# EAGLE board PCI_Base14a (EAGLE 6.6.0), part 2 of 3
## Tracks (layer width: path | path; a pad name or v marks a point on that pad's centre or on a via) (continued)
CLK2  (via drill 0.3) (continued)
  Top 0.254: v31.75,124.45 32.07,124.45 32.07,114.45 31.75,114.13 31.75,109.68 30.48,108.41 30.48,107.62 30.32,107.46 30.32,81.9 29.69,81.27 29.69,72.38 v30,72.06 | v33.34,72.06 34.13,71.27 34.13,64.76 33.5,64.12 v33.5,59.36 | v68.58,60 68.9,60.31 68.9,69.2 v68.58,69.52 | v107.63,69.84 107.31,70.16 107.31,70.31 107,70.63 107,73.97 106.36,74.6 106.36,77.78 106.04,78.09 106.04,86.67 106.84,87.46 106.84,113.81 v107.16,114.13 | v103.82,114.13 104.14,114.45 104.14,138.89 v103.82,139.21
  Bottom 0.152: X6.J3-A27 arc-90 X6.J3-A27 100.33,139.21
  Bottom 0.254: v31.75,124.45 33.18,124.45 34.13,125.4 36.04,125.4 36.51,125.88 37.31,125.88 X2.B16 | v33.34,72.06 v30,72.06 | v33.5,59.36 33.81,59.68 34.92,59.68 35.56,60.31 36.67,60.31 36.99,60.63 46.35,60.63 47.47,59.52 48.74,59.52 49.21,60 v68.58,60 | v68.58,69.52 68.9,69.2 71.91,69.2 72.55,69.84 75.41,69.84 75.72,70.16 83.18,70.16 83.5,69.84 v107.63,69.84 | v103.82,114.13 v107.16,114.13 | 100.33,139.21 v103.82,139.21
CLK3  (via drill 0.3)
  Top 0.254: v7.46,126.04 7.46,127.15 8.1,127.78 8.1,142.7 7.78,143.02 7.78,150.8 7.46,151.12 v7.3,151.12 | v24.92,152.07 24.61,152.39 24.61,158.9 24.92,159.21 v24.92,167.15 | v73.34,166.68 73.34,156.36 73.66,156.04 73.66,150.17 73.34,149.85 73.34,147.15 74.93,145.56 74.93,142.39 73.82,141.28 v73.82,140.16
  Bottom 0.152: X6.J3-C27 89.38,139.21 88.74,139.93 88.15,140.2 81.36,140.2
  Bottom 0.254: v7.46,126.04 8.57,126.04 8.89,126.35 13.81,126.35 14.29,125.88 16.67,125.88 X3.B16 | v7.3,151.12 7.62,151.44 7.94,151.44 8.25,151.75 11.27,151.75 11.59,152.07 13.33,152.07 13.65,152.39 24.61,152.39 v24.92,152.07 | v24.92,167.15 26.51,167.15 26.83,166.83 27.62,166.83 27.94,166.52 48.58,166.52 49.21,167.15 49.85,167.15 50.96,166.04 63.82,166.04 64.45,166.68 v73.34,166.68 | v73.82,140.16 74.93,140.16 75.25,140.48 80.96,140.48 81.36,140.2
DEVSEL#  (via drill 0.3)
  Top 0.254: v85.25,109.21 84.93,108.89 84.93,106.67 84.61,106.35 84.61,101.11 84.93,100.79 84.93,89.84 85.25,89.52 85.25,84.13 84.14,83.01 v84.14,73.01 | v80.96,73.01 81.28,73.01 81.28,65.23 80.64,64.6 80.64,63.96 81.76,62.85 81.76,55.07 81.44,54.76 v81.44,53.65 | v29.37,58.09 v29.37,53.65 | v8.57,58.09 8.89,58.09 8.89,65.39 9.21,65.71 9.21,86.19 v8.89,86.51 | v20.48,87.94 20.64,88.09 20.64,88.25 21.43,89.05 22.38,89.05 23.34,90 23.65,90 23.97,90.32 24.92,90.32 25.4,90.79 v25.72,90.79 | v29.05,90.79 29.37,91.11 29.37,99.21 v29.05,99.52
  Bottom 0.152: X6.J3-D12 v85.25,109.21
  Bottom 0.254: 29.05,99.21 26.19,99.21 24.92,100.48 23.97,100.48 22.7,99.21 19.37,99.21 X3.B37 | 29.05,99.21 39.85,99.21 X2.B37 40,99.21 43.34,99.21 44.61,100.48 45.56,100.48 46.83,99.21 60.48,99.21 X1.B37 | v80.96,73.01 v84.14,73.01 | v81.44,53.65 81.12,53.96 39.69,53.96 39.37,53.65 v29.37,53.65 | v29.37,58.09 29.05,57.77 13.02,57.77 12.7,58.09 v8.57,58.09 | v8.89,86.51 17.3,86.51 18.57,87.78 20,87.78 20.16,87.94 v20.48,87.94 | v29.05,90.79 v25.72,90.79 | 29.05,99.21 v29.05,99.52
FRAME#  (via drill 0.3)
  Top 0.254: v10,101.43 10,98.57 10.32,98.25 10.32,88.25 10.64,87.94 10.64,64.76 10.32,64.44 10.32,57.14 10,56.82 v10,55.71 | v50.64,56.03 v50.64,61.27 50.64,72.22 v50.32,72.54 | v93.66,61.9 93.98,62.22 93.98,76.51 94.3,76.82 94.3,80.63 93.98,80.95 93.98,81.9 v94.14,82.06 | v99.22,82.06 98.9,82.38 98.9,88.41 99.22,88.73 99.22,89.36 98.9,89.68 98.9,97.62 99.22,97.94 99.22,98.57 98.11,99.68 98.11,109.53 98.42,109.84 v98.42,111.27 | v55.72,97.46 55.88,97.46 57.63,99.21 58.42,99.21 58.74,99.52 59.21,99.52 60.17,100.48 60.96,100.48 61.59,101.11 62.07,101.11 63.18,102.22 63.18,103.02 X1.A34 | v52.07,97.46 51.75,97.14 51.75,89.68 51.43,89.36 51.43,84.28 51.59,84.13 51.59,72.85 v51.91,72.54
  Bottom 0.152: X6.J3-A13 arc-90 93.42,111.27 v98.42,111.27
  Bottom 0.254: v10,101.43 16.03,101.43 16.35,101.75 17.3,101.75 18.57,103.02 21.75,103.02 X3.A34 21.91,103.02 24.92,103.02 25.24,102.7 26.03,102.7 26.51,102.22 36.51,102.22 36.99,101.75 37.94,101.75 39.21,103.02 42.39,103.02 X2.A34 | v10,55.71 11.11,55.71 11.43,56.03 13.02,56.03 13.33,56.34 31.27,56.34 31.59,56.66 45.88,56.66 46.2,56.34 49.05,56.34 49.37,56.03 v50.64,56.03 | v50.64,61.27 50.96,60.95 67.63,60.95 68.26,61.58 78.74,61.58 79.06,61.27 85.41,61.27 85.72,61.58 93.34,61.58 v93.66,61.9 | v99.22,82.06 v94.14,82.06 | v52.07,97.46 v55.72,97.46 | v50.32,72.54 v51.91,72.54
GND  (via drill 0.3)
  Top 0.254: X2.B57 40,73.97 40,74.44 40.16,74.6 42.54,74.6 42.54,75.08 X2.A56 42.54,75.24 42.54,75.87 43.81,77.14 43.81,80.63 43.66,80.79 43.66,82.7 43.5,82.86 43.5,83.17 42.54,84.13 42.54,85.24 X2.A48 | v35.88,83.97 v35.88,87.78 v35.88,97.94 v35.88,101.43 v35.88,103.02 v35.88,110.64 v35.88,118.26 | X3.A42 21.91,93.02 21.91,93.81 22.22,94.13 22.38,94.13 23.18,94.92 23.18,97.14 24.45,98.41 24.45,99.21 X3.A37 24.45,99.37 24.45,101.75 X3.A35 | v40.96,110.48 42.54,108.89 42.54,108.26 X2.A30 | X2.A24 42.54,115.88 42.54,116.51 v40.96,118.1 41.12,118.1 41.12,118.89 41.27,119.05 41.27,121.27 42.54,122.54 42.54,123.34 X2.A18 | X2.B17 40,124.77 40,127.15 X2.B15 40,127.31 40,129.69 X2.B13 | 40,130.32 37.62,130.32 37.46,130.48 37.46,130.96 X2.B12 | 40,130.32 40,129.85 X2.B13 | 40,130.32 40,130.64 42.07,130.64 42.39,130.96 X2.A12 | 40,130.32 X2.B13 | C3.2 51.12,143.5 v51.12,139.85 51.12,137.47 C4.2 51.12,137.31 v51.12,130.96 v51.12,129.69 | v59.05,140.16 60.64,141.75 60.64,142.39 X1.B3 | X1.B13 60.64,129.69 60.64,127.31 X1.B15 60.64,127.15 60.64,124.77 X1.B17 60.64,124.61 60.64,123.65 62.07,123.65 62.23,123.5 63.02,123.5 X1.A18 | v38.1,145.72 38.42,145.4 38.42,144.77 40,143.18 40,142.55 X2.B3 | v29.53,145.72 29.53,143.66 C1.2 29.53,143.5 29.53,137.47 C2.2 29.53,137.31 29.53,132.86 29.05,132.39 29.05,130.96 | X3.B17 19.37,124.77 19.37,127.15 X3.B15 19.37,127.31 19.37,129.69 X3.B13 | v15.24,130.96 v15.24,142.39 | v29.05,129.69 29.05,130.96 | v15.24,74.12 15.24,77.93 14.92,78.25 14.92,83.65 v15.24,83.97 v15.24,87.78 15.24,91.9 14.92,92.22 14.92,97.62 v15.24,97.94 v15.24,103.02 v15.24,110.64 v15.24,118.26 v15.24,124.61
  Top 0.254: v18.26,108.41 16.83,109.84 16.83,110.64 X3.B28 | 29.05,130.96 v29.37,130.96 | v76.83,35.07 76.83,38.09 C12.2 | 89.06,30.94 X7.16 89.06,30.79 | 89.06,34.91 X7.17 | 89.06,26.66 X7.15 | 95.57,8.4 JP4.1 | 89.06,18.09 X7.13 | v78.1,60.31 C8.- | v75.56,60.31 75.56,64.12 C7.+ | C10.- v86.36,60.31 86.36,64.12 C9.- v86.36,66.66 | v64.77,66.66 64.77,67.93 64.45,68.25 64.45,73.01 63.18,74.28 63.18,75.08 X1.A56 | X1.B46 58.1,87.78 58.1,86.98 60.64,84.44 60.64,84.28 60.48,84.13 X1.B49 | v47.47,98.41 47.15,98.1 47.15,92.86 v47.47,92.86 47.47,92.54 47.62,92.38 47.62,91.27 48.1,90.79 48.1,88.89 48.42,88.57 48.42,88.41 v48.58,88.25 | X2.A35 45.08,101.75 45.08,99.37 X2.A37 | X1.A42 63.18,93.02 63.18,93.81 64.45,95.08 64.45,97.14 65.72,98.41 65.72,99.21 X1.A37 65.72,99.37 65.72,101.75 X1.A35 | v56.51,118.26 v56.51,110.64 | v61.59,118.1 63.18,116.51 63.18,115.88 X1.A24 | 71.12,108.41 71.12,115.56 C16.2 | 71.12,108.41 71.12,108.1 C15.2 | 71.12,108.41 v69.85,108.41 | 71.12,108.41 C15.2 | v61.59,110.48 63.18,108.89 63.18,108.26 X1.A30 | C15.2 71.12,107.94 v71.12,101.75 v71.12,100 | H1.B3,3 87.79,153.18 87.79,147.31 87.31,146.83 87.31,145.24 X6.J3-D30 | C17.2 96.52,79.52 96.52,81.11 96.04,81.59 96.04,86.82 v96.36,87.14 96.04,86.98 96.04,91.75 v96.36,92.06 96.04,91.9 96.04,94.92 v96.36,95.24 | 83.66,100.48 v83.66,107.3 v83.62,110.24 83.94,110.56 83.98,114.92 v83.66,115.24 v83.7,118.14 83.82,118.26 v83.82,125.24 84.14,125.24 84.14,129.85 v83.9,130.2 84.14,130 84.14,133.97 84.45,134.29 v84.45,135.24 v84.45,138.26 83.82,138.89 v83.82,145.24 | v94.77,105.24 v94.77,112.22 v94.77,113.18
  Top 0.254: v94.77,122.23 v94.77,125.24 95.09,125.56 v95.09,132.07 v95.09,133.18 94.77,133.5 94.77,136.51 95.09,136.83 95.09,140.96 v94.77,141.28 | C5.2 71.44,143.5 71.44,137.47 C6.2 71.44,137.31 v71.44,135.08 v71.44,129.69 | v83.66,95.24 83.34,95.56 83.34,100.16 83.66,100.48 | 83.66,100.48 v83.7,100.2 | v93.34,79.52 93.34,87.14 X6.J3-A1 | v87.79,64.28 87.79,79.52 H2.B3,3 | v80.17,35.07 80.49,35.39 v80.49,57.93
  Top 0.813: 89.06,34.91 89.06,30.94 | 89.06,26.66 89.06,30.79 | v95.57,16.34 95.57,8.4 | 89.06,18.09 v89.06,16.34 | v86.36,18.24 v86.36,26.66 | v76.68,10.94 v76.68,18.24
  Bottom 0.152: X6.J3-A1 93.36,87.14 v96.36,87.14 101.6,87.14 | X6.J3-D30 87.36,145.24 v83.82,145.24 80.01,145.24 | X6.J3-D27 87.36,139.05 83.66,139.05 80.01,139.05 | X6.J3-C26 88.8,138.1 arc90 88.65,138.26 v84.45,138.26 83.66,138.26 81.44,138.26 | X6.J3-D20 87.36,125.24 | 87.36,125.24 87.63,125.24 | 87.36,125.24 v83.82,125.24 80.01,125.24 | X6.J3-D11 87.36,107.3 v83.66,107.3 79.85,107.3 | X6.J3-D5 87.36,95.24 v83.66,95.24 80.01,95.24 | X6.J3-C4 88.57,94.29 83.66,94.13 81.28,94.13 | X6.J3-A28 arc-90 93.43,141.28 v94.77,141.28 100.17,141.28 | X6.J3-A20 arc90 93.49,125.08 100.17,125.08 | X6.J3-A14 arc90 93.55,113.02 100.33,113.02 | X6.J3-A10 93.36,105.18 arc90 93.61,104.92 97,104.92 100.33,104.92 | X6.J3-A5 arc-90 93.39,95.24 v96.36,95.24 100.17,95.24 | X6.J3-C22 89.36,129.91 arc66 88.49,130.14 arc24 88.31,130.2 v83.9,130.2 | v83.9,130.2 81.28,130.16 | X6.J3-C16 89.36,117.84 arc90 88.47,118.22 v83.7,118.14 81.28,118.1 | X6.J3-C12 89.36,110.07 arc19 88.47,110.19 arc71 88.51,110.2 v83.62,110.24 81.28,110.32 | X6.J3-C7 89.36,99.91 arc90 88.47,100.2 v83.7,100.2 81.28,100.16 | X6.J3-D15 arc90 87.33,115.24 v83.66,115.24 80.01,115.24 | X6.J3-B18 91.36,121.97 arc-90 91.61,122.23 v94.77,122.23 101.6,122.23 | X6.J3-B23 91.36,131.81 arc-90 91.61,132.07 92.23,132.07 92.23,132.31 94.06,132.23 94.06,132.07 v95.09,132.07 101.6,132.07 | X6.J3-A24 arc90 93.39,133.18 v95.09,133.18 100.33,133.18 | X6.J3-D25 arc90 87.33,135.24 v84.45,135.24 80.17,135.24 | X6.J3-B9 92.47,103.87 arc-90 92.72,104.29 97,104.29 101.6,104.13 | X6.J3-B13 92.23,111.97 arc-90 92.65,112.22 v94.77,112.22 101.44,112.14
  Bottom 0.152: X6.J3-B3 91.36,91.81 arc-56 91.47,92.02 arc-34 91.61,92.22 94.69,92.22 94.69,92.06 v96.36,92.06 101.6,92.06 | 86.36,129.53 86.27,129.53 | 78.42,129.85 78.5,129.81 | 78.9,130 78.91,129.98 | 67.47,128.58 67.46,128.6 | 66.52,128.89 66.51,128.82 | 65.88,129.58 65.88,129.53 X1.A13 65.88,129.69 | 80.01,131.12 80.01,131.15 | 77.47,131.75 77.47,131.72 | 77.31,131.75 77.31,131.72 | 80.64,131.75 80.64,131.72 | 72.55,129.21 72.54,129.27 | 72.87,129.53 72.91,129.48 | 76.68,129.37 76.69,129.47 | 75.25,129.21 75.25,129.24 | 66.83,129.21 66.87,129.18 | 86.84,130.16 86.83,130.21 | 80.17,129.53 80.27,129.51 | 78.1,129.21 78.1,129.24 | 69.21,128.1 69.21,128.13 | 69.53,128.1 69.45,128.13 | 67.79,128.58 67.79,128.68 | 83.66,130.32 v83.9,130.2 | 80.33,131.12 80.33,131.22 | 77.79,130.64 77.84,130.74 | 77.63,130.64 77.59,130.72 | 72.71,130.8 72.66,130.69 | 72.87,130.8 72.81,130.77 | 73.66,130.48 73.66,130.51 | 78.26,131.75 78.26,131.72 | 80.01,131.75 80.01,131.72 | 72.23,130.64 72.24,130.74 72.23,130.8 | 71.6,130 v71.44,129.69 71.6,129.85 | 74.61,129.53 74.61,129.5 | 76.36,129.53 76.36,129.5 | 72.39,130.8 72.39,130.74 | 67.63,128.58 67.64,128.68 | 83.34,130.48 83.35,130.45 | 86.68,130.48 86.62,130.42 | 69.53,128.26 69.54,128.36 | 66.83,128.42 66.87,128.46 | 73.98,130.96 73.97,130.86 | 80.96,130.16 80.95,130.06 | 80.64,129.85 80.66,129.82 | 78.9,131.27 79,131.26 | 70.33,130.8 70.33,130.77 | 72.07,130.8 72.12,130.69 | 73.5,130.48 73.5,130.51 | 73.98,131.75 73.97,131.69 | 70.64,130.8 70.64,130.77 | S2.2
  Bottom 0.254: v35.88,87.78 37.31,87.78 X2.B46 | v35.88,83.97 35.88,83.65 37.46,83.65 37.78,83.97 39.69,83.97 39.85,84.13 | 39.85,84.13 40.16,84.44 40.64,84.44 41.43,85.24 42.39,85.24 X2.A48 | 39.85,84.13 X2.B49 | v35.88,97.94 37.31,97.94 X2.B38 | v35.88,103.02 37.31,103.02 X2.B34 | v35.88,110.64 37.31,110.64 X2.B28 37.46,110.64 40.48,110.64 40.64,110.48 v40.96,110.48 | v35.88,118.26 37.31,118.26 X2.B22 37.46,118.26 40.48,118.26 40.64,118.1 v40.96,118.1 | v35.88,101.43 35.56,101.75 24.45,101.75 X3.A35 | X2.A12 42.54,130.96 43.18,130.96 44.45,129.69 44.93,129.69 X2.A13 45.08,129.69 v51.12,129.69 | X2.A18 42.39,123.34 41.91,123.34 40.64,124.61 40,124.61 X2.B17 | v59.05,140.16 58.74,140.16 58.42,139.85 v51.12,139.85 | 58.98,130.56 59.85,129.69 60.48,129.69 X1.B13 | 58.98,130.56 58.58,130.96 58.1,130.96 X1.B12 57.94,130.96 v51.12,130.96 | 58.98,130.56 59.05,130.64 61.59,130.64 61.91,130.96 63.02,130.96 X1.A12 63.18,130.96 63.98,130.96 64.29,130.64 64.77,130.64 65.56,129.85 X1.A13 65.72,129.69 65.88,129.69 v71.44,129.69 | v38.1,145.72 37.78,145.4 29.84,145.4 v29.53,145.72 | X3.A18 21.75,123.5 20.95,124.29 20.48,124.29 20.16,124.61 19.37,124.61 X3.B17 19.21,124.61 v15.24,124.61 | 17.7,130.56 18.57,129.69 19.21,129.69 X3.B13 | 17.7,130.56 17.3,130.96 16.83,130.96 X3.B12 16.67,130.96 v15.24,130.96 | v15.24,142.39 19.21,142.39 X3.B3 | 17.7,130.56 17.78,130.64 20.48,130.64 20.8,130.96 21.75,130.96 X3.A12 21.91,130.96 22.54,130.96 23.81,129.69 24.29,129.69 X3.A13 24.45,129.69 v29.05,129.69 | X3.A56 21.75,75.08 21.11,75.08 19.84,73.81 19.37,73.81 X3.B57 19.21,73.81 16.35,73.81 16.03,74.12 v15.24,74.12
  Bottom 0.254: v15.24,87.78 16.67,87.78 X3.B46 | v15.24,83.97 15.24,83.65 16.99,83.65 17.3,83.97 19.05,83.97 19.21,84.13 X3.B49 19.37,84.13 19.68,84.44 20,84.44 20.8,85.24 21.75,85.24 X3.A48 | v15.24,97.94 16.67,97.94 X3.B38 | v15.24,103.02 16.67,103.02 X3.B34 | v15.24,110.64 16.67,110.64 X3.B28 | v15.24,118.26 16.67,118.26 X3.B22 16.83,118.26 17.78,118.26 17.78,116.83 18.89,115.72 21.75,115.72 X3.A24 | v18.26,108.41 18.57,108.41 18.89,108.1 21.75,108.1 X3.A30 | v29.37,130.96 37.31,130.96 X2.B12 | v76.83,35.07 v80.17,35.07 83.5,35.07 X7.7 83.66,35.07 | 83.66,26.66 X7.5 | 89.06,26.66 X7.15 | 89.06,35.07 X7.17 | 83.66,18.24 X7.3 83.5,18.24 | 89.06,18.24 X7.13 | 74.93,10.94 X5.1 | v75.56,60.31 v78.1,60.31 v86.36,60.31 | X1.B57 60.64,73.81 61.44,73.81 62.71,75.08 63.02,75.08 X1.A56 | v64.77,66.66 65.09,66.35 76.99,66.35 77.31,66.66 v86.36,66.66 | X1.A48 63.02,85.24 61.75,85.24 60.8,84.28 60.64,84.28 60.48,84.13 X1.B49 | v47.47,92.86 42.54,92.86 X2.A42 | X2.A37 45.08,99.21 46.04,99.21 46.51,98.73 47.15,98.73 v47.47,98.41 47.31,98.73 55.56,98.73 56.36,97.94 57.94,97.94 X1.B38 58.1,97.94 60.96,97.94 61.59,98.57 62.07,98.57 62.71,99.21 65.56,99.21 X1.A37 | v48.58,88.25 48.89,88.57 55.56,88.57 56.36,87.78 57.94,87.78 X1.B46 | X1.B34 58.1,103.02 61.12,103.02 61.75,102.38 62.07,102.38 62.71,101.75 65.56,101.75 X1.A35 65.72,101.75 v71.12,101.75 | v56.51,110.64 57.94,110.64 X1.B28 58.1,110.64 61.12,110.64 61.28,110.48 v61.59,110.48 | v56.51,118.26 57.94,118.26 X1.B22 58.1,118.26 61.12,118.26 61.28,118.1 v61.59,118.1 | v69.85,108.41 66.36,108.41 66.04,108.1 63.18,108.1 X1.A30 | 83.66,94.13 v83.66,95.24
  Bottom 0.254: X6.J3-C4 89.38,93.17 89.85,93.17 90.96,92.06 91.44,92.06 91.47,92.02 | 97,104.29 97,104.92 | v94.77,105.24 93.5,105.24 X6.J3-A10 | v94.77,113.18 93.5,113.18 X6.J3-A14 | X6.J3-B13 91.28,111.11 90.96,110.8 90.49,110.8 89.85,110.16 89.38,110.16 88.47,110.19 | v94.77,125.24 93.5,125.24 X6.J3-A20 | 83.66,138.26 83.66,139.05 | v71.44,135.08 71.75,134.77 79.69,134.77 80.17,135.24 | X6.J3-B23 91.28,131.12 90.96,130.8 90.49,130.8 89.85,130.16 89.22,130.16 88.49,130.14 | v93.34,79.52 H2.B3,3 | v71.12,100 74.14,100 74.45,99.68 80.8,99.68 81.28,100.16 | v87.79,64.28 86.52,64.28 C9.- | v80.49,57.93 78.26,57.93 C8.- | S2.2 109.38,8.4 111.12,10.15 111.12,119.76 110.65,120.24 108.97,120.24 JP5.2
  Bottom 0.813: 89.06,26.66 v86.36,26.66 83.66,26.66 | 89.06,35.07 83.66,35.07 | v89.06,16.34 v95.57,16.34 | 89.06,18.24 v86.36,18.24 83.66,18.24 | v76.68,18.24 83.5,18.24 | 74.93,10.94 v76.68,10.94
  other vias: 27.94,100.95 27.78,107.94 27.62,112.86 9.84,106.19 101.28,111.27
  pour Top (isolate 0.254): -1.27,188.74 115.57,188.74 115.57,-1.76 -1.27,-1.76
  pour Bottom (isolate 0.254): -1.27,188.74 115.57,188.74 115.57,-1.76 -1.27,-1.76
GNT1#  (via drill 0.3)
  Top 0.254: v79.53,146.36 v79.53,124.61 | v88.42,146.2 91.44,149.21 v91.44,150.8 | v102.08,152.07 102.08,148.26 101.12,147.31 101.12,135.4 v101.44,135.08
  Bottom 0.152: X6.J3-A25 arc90 93.49,135.08 100.17,135.08
  Bottom 0.254: v79.53,124.61 65.72,124.61 X1.A17 | v79.53,146.36 87.79,146.36 87.95,146.2 v88.42,146.2 | v91.44,150.8 96.84,150.8 97.47,151.44 99.06,151.44 99.38,151.75 100.17,151.75 100.49,152.07 v102.08,152.07 | 100.17,135.08 v101.44,135.08
GNT2#  (via drill 0.3)
  Top 0.254: v55.56,124.61 55.56,125.88 55.24,126.19 55.24,133.81 55.88,134.45 57.31,134.45 57.63,134.77 58.42,134.77 v59.53,135.88 | v78.74,136.2 v78.74,133.5
  Bottom 0.152: X6.J3-C25 89.36,136.05 arc90 89.22,136.2 81.28,136.2
  Bottom 0.254: v55.56,124.61 45.08,124.61 X2.A17 | v59.53,135.88 60.01,135.88 60.17,136.04 61.12,136.04 61.75,135.4 62.07,135.4 62.71,134.77 63.66,134.77 64.29,134.13 64.61,134.13 65.25,133.5 67.63,133.5 67.94,133.81 78.42,133.81 v78.74,133.5 | 81.28,136.2 v78.74,136.2
GNT3#  (via drill 0.3)
  Top 0.254: v27.62,124.45 27.3,124.77 27.3,130.8 27.62,131.12 27.62,131.75 27.15,132.23 27.15,139.85 26.99,140.01 26.99,149.21 27.78,150.01 27.78,150.96 26.99,151.75 26.99,157.31 27.3,157.63 27.3,162.07 26.99,162.39 v26.99,165.56 | v64.77,165.88 64.93,165.72 64.93,165.09 65.25,164.77 65.25,157.94 66.04,157.15 v66.04,146.67
  Bottom 0.152: X6.J3-C30 89.36,146.83 80.17,146.83 80.01,146.83
  Bottom 0.254: v27.62,124.45 27.46,124.61 24.45,124.61 X3.A17 | v26.99,165.56 64.45,165.56 v64.77,165.88 | v66.04,146.67 78.74,146.67 79.22,147.15 79.85,147.15 80.17,146.83
IDSEL1  (via drill 0.3)
  Top 0.254: v69.06,113.81 68.74,113.81 68.74,118.26 69.06,118.57 69.06,121.91 v69.37,122.23
  Bottom 0.152: X6.J3-C18 89.36,121.97 arc90 89.11,122.23 81.28,122.23
  Bottom 0.254: v69.06,113.81 66.67,113.81 66.04,113.18 63.18,113.18 X1.A26 | 81.28,122.23 v69.37,122.23
IDSEL2  (via drill 0.3)
  Top 0.254: v47.47,120.32 47.15,120 47.15,116.51 46.67,116.03 46.67,114.29 45.56,113.18 44.61,113.18 43.81,113.97 42.7,113.97 42.54,113.81 42.54,113.34 X2.A26 | v52.23,136.04 v52.23,120.32 | v64.13,137.62 64.13,137.94 64.45,138.26 64.45,140.32 65.25,141.12 66.04,141.12 66.36,141.43 v66.67,141.43 | v72.23,138.74 v72.23,141.59 | v72.55,136.04 72.55,130.96 73.18,130.32 73.18,129.69 72.87,129.37 72.87,121.75 v73.18,121.43
  Bottom 0.152: X6.J3-D18 87.36,121.27 80.01,121.27
  Bottom 0.254: v47.47,120.32 47.78,120 51.91,120 v52.23,120.32 | v52.23,136.04 53.02,136.83 57.15,136.83 57.63,137.31 58.42,137.31 59.05,137.94 59.53,137.94 60.17,138.58 61.12,138.58 61.75,137.94 62.07,137.94 62.71,137.31 63.5,137.31 63.82,137.62 v64.13,137.62 | v66.67,141.43 67.15,141.43 67.31,141.59 v72.23,141.59 | v72.23,138.74 72.55,138.42 v72.55,136.04 | v73.18,121.43 73.5,121.75 79.53,121.75 80.01,121.27
IDSEL3  (via drill 0.3)
  Top 0.254: v23.02,114.76 22.86,114.76 21.91,113.81 21.91,113.34 X3.A26 | v34.29,113.65 34.29,120.64 34.61,120.96 34.61,127.94 33.34,129.21 33.34,134.29 33.5,134.45 33.5,135.08 33.18,135.4 33.18,137.78 34.13,138.74 34.13,142.07 34.45,142.39 34.45,147.31 33.81,147.94 33.81,153.66 34.29,154.13 v34.29,164.45 | v65.72,165.41 65.72,158.26 66.52,157.47 66.52,147.94 67.47,146.99 67.47,142.7 v67.15,142.39 | v86.04,141.59 85.72,141.28 85.72,134.93 86.2,134.45 86.2,132.54 85.57,131.91 85.57,125.24 87.31,123.5 87.31,123.34 X6.J3-D19
  Bottom 0.152: X6.J3-D19 87.36,123.18
  Bottom 0.254: v23.02,114.76 23.97,115.72 25.88,115.72 27.62,113.97 33.97,113.97 v34.29,113.65 | v34.29,164.45 34.61,164.14 36.35,164.14 36.67,163.82 42.54,163.82 42.86,164.14 45.24,164.14 46.2,165.09 65.4,165.09 v65.72,165.41 | v67.15,142.39 67.47,142.07 71.6,142.07 72.07,142.55 80.49,142.55 81.6,141.43 85.88,141.43 v86.04,141.59
INTA#  (via drill 0.3)
  Top 0.254: v23.02,144.61 23.02,144.29 23.18,144.13 23.18,140.64 21.91,139.37 21.91,138.74 X3.A6 | v24.13,159.53 v24.13,146.36 | v66.52,158.9 66.67,158.74 66.67,158.1 66.99,157.79 66.99,148.26 67.94,147.31 67.94,141.12 v67.63,140.8 | v45.88,143.66 44.61,143.66 43.81,142.86 43.81,140.64 42.54,139.37 42.54,138.74 X2.A6 | v56.04,144.13 55.72,144.45 55.72,152.07 56.04,152.39 56.04,153.18 56.36,153.5 v56.36,158.9 | v97.15,159.21 v97.15,144.21
  Bottom 0.152: v97.15,144.21 92.31,144.21 X6.J3-B29
  Bottom 0.254: v23.02,144.61 23.02,145.24 v24.13,146.36 | v24.13,159.53 24.45,159.21 33.65,159.21 34.29,158.58 56.36,158.58 | 56.36,158.58 66.2,158.58 v66.52,158.9 66.83,159.21 v97.15,159.21 | v67.63,140.8 68.1,140.32 68.1,139.05 66.52,139.05 66.04,138.58 63.18,138.58 X1.A6 | v45.88,143.66 46.67,144.45 55.72,144.45 v56.04,144.13 | 56.36,158.58 v56.36,158.9
INTB#  (via drill 0.3)
  Top 0.254: X1.B7 60.64,137.47 60.64,137.62 58.74,137.62 58.42,137.31 57.63,137.31 56.51,138.42 v56.51,138.58 56.2,138.89 56.2,143.18 56.83,143.82 56.83,144.13 57.31,144.61 v57.31,146.51 | v70.96,144.93 70.64,145.24 70.64,150.01 70.96,150.32 70.96,161.75 71.28,162.07 v71.28,163.82 | v52.23,146.51 v52.23,163.82
  Bottom 0.152: X6.J3-C29 88.65,143.8 arc90 87.84,144.21 85.09,144.21 85.09,144.29 81.44,144.37
  Bottom 0.254: v56.51,138.58 56.2,138.89 52.07,138.89 51.75,138.58 44.61,138.58 43.97,137.94 43.66,137.94 43.02,137.31 40,137.31 X2.B7 39.85,137.31 36.99,137.31 36.51,136.83 33.65,136.83 32.07,135.24 28.26,135.24 24.92,138.58 23.97,138.58 23.34,137.94 23.02,137.94 22.38,137.31 19.37,137.31 X3.B7 | 81.44,144.37 80.96,144.77 77.79,144.77 77.47,145.09 73.18,145.09 72.87,144.77 71.12,144.77 v70.96,144.93 | v71.28,163.82 70.96,164.14 52.55,164.14 v52.23,163.82 | v57.31,146.51 v52.23,146.51
INTC#  (via drill 0.3)
  Top 0.254: v69.69,137.31 69.37,137.62 69.37,142.7 v69.69,143.02 69.37,142.86 69.37,147.63 69.69,147.94 v69.69,150.96 | v26.03,150.17 26.03,139.69 24.92,138.58 24.76,138.58 24.45,138.26 24.45,137.47 X3.A7 | v46.67,150.17 46.67,139.69 45.08,138.1 45.08,137.47 X2.A7
  Bottom 0.152: X6.J3-D29 87.36,143.02 80.01,143.02
  Bottom 0.254: v69.69,137.31 65.72,137.31 X1.A7 | 80.01,143.02 v69.69,143.02 | v26.03,150.17 26.35,149.85 43.02,149.85 43.34,150.17 v46.67,150.17 46.99,149.85 51.59,149.85 52.7,150.96 53.34,150.96 53.97,150.32 63.34,150.32 63.66,150.64 69.37,150.64 v69.69,150.96
INTD#  (via drill 0.3)
  Top 0.254: v14.45,136.04 14.76,136.35 14.76,141.75 14.45,142.07 v14.45,149.37 | v35.08,136.04 35.08,141.43 35.4,141.75 35.4,148.26 v35.08,148.58 35.4,148.42 35.4,151.59 35.08,151.91 v35.08,153.02 | v55.09,136.04 54.77,136.35 v54.77,153.02 | v103.5,158.42 v103.5,142.23 | v75.88,153.18 v75.88,157.47
  Bottom 0.152: 101.6,142.15 92.47,142.23 X6.J3-B28
  Bottom 0.254: v14.45,136.04 16.67,136.04 X3.B8 | v14.45,149.37 21.91,149.37 22.7,148.58 23.34,148.58 23.65,148.9 34.77,148.9 v35.08,148.58 | v35.08,136.04 37.31,136.04 X2.B8 | v55.09,136.04 57.94,136.04 X1.B8 | v35.08,153.02 36.19,153.02 36.51,152.71 47.62,152.71 47.94,153.02 v54.77,153.02 55.88,153.02 56.04,153.18 57.78,153.18 58.42,153.82 71.91,153.82 72.23,153.5 75.88,153.5 v75.88,153.18 | v103.5,142.23 101.6,142.15 | v103.5,158.42 96.84,158.42 96.52,158.74 78.58,158.74 77.31,157.47 v75.88,157.47
IRDY#  (via drill 0.3)
  Top 0.254: v17.94,103.97 19.37,102.54 19.37,101.91 X3.B35 | v9.21,103.97 9.21,101.11 9.52,100.79 9.52,98.25 9.84,97.94 9.84,87.94 10.16,87.62 10.16,65.08 9.84,64.76 9.84,57.46 9.52,57.14 9.52,56.34 9.21,56.03 v9.21,54.92 | v51.43,55.23 51.43,62.22 51.12,62.54 51.12,83.81 50.96,83.97 50.96,89.68 51.28,90 v51.28,102.06 | v82.87,112.22 82.87,106.99 83.18,106.67 83.18,100.79 82.87,100.48 82.87,92.86 83.18,92.54 83.18,76.98 v82.87,76.66 | v79.53,67.46 v79.53,76.35 | v65.72,67.14 65.56,66.98 65.56,66.35 65.25,66.03 65.25,58.88 65.56,58.57 v65.56,55.23
  Bottom 0.152: X6.J3-C13 89.36,111.97 arc90 89.11,112.22 v82.87,112.22
  Bottom 0.254: v17.94,103.97 17.62,103.97 17.3,104.29 16.35,104.29 16.03,103.97 v9.21,103.97 | v9.21,54.92 10.32,54.92 10.64,55.23 11.43,55.23 11.75,55.55 13.33,55.55 13.65,55.87 31.59,55.87 31.91,56.19 45.56,56.19 45.88,55.87 48.74,55.87 49.05,55.55 50.01,55.55 50.32,55.23 v51.43,55.23 51.75,54.92 65.25,54.92 v65.56,55.23 | X1.B35 60.48,101.75 51.59,101.75 v51.28,102.06 51.43,101.75 48.58,101.75 48.42,101.91 46.67,101.91 45.56,103.02 44.61,103.02 44.29,102.7 43.97,102.7 43.02,101.75 40,101.75 X2.B35 | v82.87,76.66 80.01,76.66 79.69,76.35 v79.53,76.35 | v79.53,67.46 79.22,67.14 76.99,67.14 76.68,66.82 66.04,66.82 v65.72,67.14
LOCK#  (via drill 0.3)
  Top 0.254: v81.6,108.26 81.28,108.57 81.28,117.62 81.76,118.1 81.76,126.19 80.96,126.99 80.96,127.62 81.28,127.94 81.28,132.07 81.6,132.39 81.6,139.53 81.91,139.85 81.91,143.66 81.6,143.97 81.6,146.2 81.28,146.51 81.28,153.02 v80.49,153.82 | v57.15,154.45 56.83,154.13 56.83,153.18 56.51,152.86 56.51,152.07 56.2,151.75 56.2,146.04 v56.51,145.72 | v53.97,145.72 54.29,145.4 54.29,142.55 53.82,142.07 v53.82,141.12 | v47.94,140.64 47.78,140.48 47.78,138.58 47.94,138.42 47.94,137.78 47.78,137.62 47.78,121.11 48.26,120.64 48.26,116.99 47.94,116.67 47.94,114.61 47.47,114.13 47.47,110.48 v47.15,110.16 | v49.21,110.16 49.53,109.84 49.53,101.59 49.21,101.27 49.21,99.05 49.53,98.73 v49.53,96.67
  Bottom 0.152: X6.J3-C11 88.57,108 arc90 88.07,108.22 v81.6,108.26 81.44,108.26
  Bottom 0.254: X3.B39 19.37,96.67 22.7,96.67 23.97,97.94 24.92,97.94 26.19,96.67 39.85,96.67 X2.B39 40,96.67 43.34,96.67 44.61,97.94 45.56,97.94 46.83,96.67 v49.53,96.67 60.48,96.67 X1.B39 | v80.49,153.82 80.17,154.13 76.83,154.13 76.52,154.45 72.87,154.45 72.55,154.77 57.47,154.77 v57.15,154.45 | v53.97,145.72 v56.51,145.72 | v53.82,141.12 53.82,141.43 48.89,141.43 48.1,140.64 v47.94,140.64 | v49.21,110.16 v47.15,110.16
N$1
  Top 0.152: R4.1 LED4.A
N$5
  Top 0.152: R1.1 LED1.A
N$6
  Top 0.152: R2.1 LED2.A
N$7
  Top 0.152: LED3.C R3.1
PAR  (via drill 0.3)
  Top 0.254: v76.52,103.18 76.83,102.86 76.83,91.9 v76.52,91.59
  Bottom 0.152: X6.J3-D9 86.72,102.86 80.33,103.02
  Bottom 0.254: X3.A43 24.45,91.59 38.26,91.59 39.53,92.86 40.48,92.86 41.75,91.59 44.93,91.59 X2.A43 45.08,91.59 58.9,91.59 60.17,90.32 60.96,90.32 62.23,91.59 65.56,91.59 X1.A43 65.72,91.59 v76.52,91.59 | v76.52,103.18 80.33,103.02
PERR#  (via drill 0.3)
  Top 0.254: v104.73,106.19 104.62,142.23 103.98,142.86 103.98,157.79 104.3,158.1 v104.3,162.07 | v35.72,155.88 v35.72,162.87 | v8.57,155.72 8.89,155.4 8.89,152.07 9.21,151.75 9.21,143.97 9.52,143.66 9.52,123.34 8.89,122.7 8.89,110.32 8.41,109.84 8.41,103.65 8.73,103.33 8.73,100.79 9.05,100.48 v9.05,95.4
  Bottom 0.152: X6.J3-B10 91.84,106.23 101.6,106.19
  Bottom 0.254: X1.B40 57.94,95.4 44.29,95.4 43.02,94.13 42.07,94.13 40.8,95.4 37.46,95.4 X2.B40 37.31,95.4 23.65,95.4 22.38,94.13 21.43,94.13 20.16,95.4 16.83,95.4 X3.B40 16.67,95.4 v9.05,95.4 | v104.73,106.19 101.6,106.19 | v104.3,162.07 98.9,162.07 98.58,161.75 95.57,161.75 94.93,161.12 61.12,161.12 60.17,162.07 46.51,162.07 45.4,163.18 43.5,163.18 43.18,162.87 v35.72,162.87 | v35.72,155.88 35.4,156.2 27.46,156.2 26.83,156.83 14.92,156.83 14.6,156.52 10.79,156.52 10.48,156.2 9.68,156.2 9.21,155.72 v8.57,155.72
PME#  (via drill 0.3)
  Top 0.254: v81.91,105.24 81.91,106.51 80.8,107.62 80.8,117.94 81.12,118.26 81.12,121.27 v79.37,123.02
  Bottom 0.152: X6.J3-D10 87.36,105.24 v81.91,105.24
  Bottom 0.254: X3.A19 24.45,122.07 38.26,122.07 39.53,123.34 40.48,123.34 41.75,122.07 44.93,122.07 X2.A19 45.08,122.07 58.9,122.07 60.17,120.8 60.96,120.8 62.23,122.07 65.56,122.07 X1.A19 65.72,122.07 67.94,122.07 68.9,123.02 69.69,123.02 70.01,122.7 79.06,122.7 v79.37,123.02
PRSTN1#  (via drill 0.3)
  Top 0.254: v32.7,134.77 32.7,138.58 31.43,139.85 31.43,143.5 C1.1 | v54.29,135.08 54.29,139.53 53.02,140.8 53.02,143.5 C3.1 53.02,143.66 v53.02,150.17 | v71.75,150.17 71.75,145.24 72.39,144.61 72.87,144.61 73.34,144.13 73.34,143.66 C5.1
  Bottom 0.254: X3.B9 19.37,134.77 22.38,134.77 23.02,135.4 23.34,135.4 23.97,136.04 24.92,136.04 26.03,134.93 26.19,134.93 26.35,134.77 v32.7,134.77 39.85,134.77 X2.B9 40,134.77 43.02,134.77 43.66,135.4 43.97,135.4 44.61,136.04 45.56,136.04 46.83,134.77 53.97,134.77 v54.29,135.08 57.31,135.08 57.63,134.77 60.48,134.77 X1.B9 | v71.75,150.17 63.98,150.17 63.66,149.85 53.34,149.85 v53.02,150.17
PRSTN2#  (via drill 0.3)
  Top 0.254: v31.43,132.23 31.43,137.31 C2.1 | v53.02,132.23 53.02,137.31 C4.1 | v73.34,131.27 73.34,137.31 C6.1
  Bottom 0.254: X3.B11 19.37,132.23 22.7,132.23 23.97,133.5 24.92,133.5 26.19,132.23 v31.43,132.23 39.85,132.23 X2.B11 40,132.23 43.34,132.23 44.61,133.5 45.56,133.5 46.83,132.23 v53.02,132.23 60.48,132.23 X1.B11 60.64,132.23 63.66,132.23 63.98,131.91 64.29,131.91 65.25,130.96 66.04,130.96 66.36,131.27 v73.34,131.27
PS_ON#  (via drill 0.3)
  Top 0.254: v90.96,49.04 v90.96,22.37 90.96,20.15 93.27,17.85 101.68,17.85 S2.1 105.41,16.02 107.95,18.56 107.95,67.77 106.84,68.89 106.84,70 106.52,70.31 106.52,73.65 105.89,74.28 105.89,77.46 105.57,77.78 105.57,86.98 106.36,87.78 v106.36,114.92 106.36,124.45 105.57,125.24 105.57,142.86 104.93,143.5 104.93,157.15 105.25,157.47 v105.41,157.47 | v76.2,104.76 76.2,109.68 75.88,110 75.88,123.5 v76.2,123.81 | v80.33,123.81 80.33,124.92 80.01,125.24 80.01,130.16 v80.33,130.48 | v78.58,130.64 77.95,131.27 77.95,138.42 78.26,138.74 78.26,143.5 v78.58,143.82 | v84.61,143.66 84.61,149.21 84.14,149.69 v84.14,157.94
  Bottom 0.152: X6.J3-C9 88.57,104.03 arc90 88.47,104.21 86.12,104.21 86.12,104.37 81.44,104.29
  Bottom 0.254: 89.22,22.37 X7.14 | v106.36,114.92 108.9,114.92 JP5.1 | 81.44,104.29 80.96,104.76 v76.2,104.76 | v80.33,123.81 v76.2,123.81 | v80.33,130.48 80.17,130.64 v78.58,130.64 | v78.58,143.82 78.9,143.5 84.45,143.5 v84.61,143.66 | v84.14,157.94 84.45,158.26 96.2,158.26 96.52,157.94 102.87,157.94 103.35,157.47 v105.41,157.47
  Bottom 0.813: 89.22,22.37 v90.96,22.37
REQ1#  (via drill 0.3)
  Top 0.254: v69.37,132.23 69.06,131.91 69.06,126.19 v69.37,125.88
  Bottom 0.152: X6.J3-C23 89.36,131.97 arc90 89.11,132.23 81.44,132.23
  Bottom 0.203: X1.B18 61.75,123.36 61.75,123.34 61.91,123.34 61.91,124.61 64.29,124.61 64.29,125.88 68.58,125.88
  Bottom 0.254: v69.37,132.23 81.44,132.23 | 68.58,125.88 v69.37,125.88
REQ2#  (via drill 0.3)
  Top 0.254: v30.64,136.04 v30.64,123.34 | v30.64,141.59 v30.64,138.74 | v32.86,141.59 32.86,152.55 32.54,152.86 32.54,154.45 30.64,156.36 30.64,160.33 30.96,160.64 30.96,161.28 30.64,161.6 v30.64,163.66 | v72.07,162.39 v72.07,164.61 | v94.3,157.47 v94.3,162.39 | v105.73,156.52 105.41,156.2 105.41,143.82 106.04,143.18 106.04,134.45 v106.36,134.13
  Bottom 0.152: X6.J3-B24 92.47,134.21 101.64,134.17
  Bottom 0.254: v30.64,123.34 37.31,123.34 X2.B18 | v30.64,138.74 v30.64,136.04 | v32.86,141.59 v30.64,141.59 | v30.64,163.66 36.04,163.66 36.35,163.34 42.86,163.34 43.18,163.66 45.56,163.66 46.51,164.61 v72.07,164.61 | v72.07,162.39 72.39,162.07 93.98,162.07 v94.3,162.39 | v94.3,157.47 102.55,157.47 103.03,156.99 104.77,156.99 105.25,156.52 v105.73,156.52 | 101.64,134.17 v106.36,134.13
REQ3#  (via drill 0.3)
  Top 0.254: v2.06,123.34 1.27,124.13 1.27,167.15 v2.06,167.95 | v74.14,162.87 v74.14,167.47 | v92.23,162.87 92.23,150.48 91.92,150.17 91.92,148.9 91.28,148.26 91.28,145.24 X6.J3-B30
  Bottom 0.152: 101.6,146.2 91.36,146.2 X6.J3-B30
  Bottom 0.254: v2.06,123.34 16.67,123.34 X3.B18 | v2.06,167.95 25.24,167.95 25.56,167.63 26.83,167.63 27.15,167.31 27.94,167.31 28.26,166.99 48.26,166.99 48.89,167.63 50.16,167.63 51.28,166.52 63.5,166.52 64.13,167.15 72.71,167.15 73.02,167.47 v74.14,167.47 | v74.14,162.87 74.45,162.55 91.92,162.55 v92.23,162.87
REQ64#  (via drill 0.3)
  Top 0.254: v61.59,65.08 61.59,67.62 63.18,69.2 63.18,70 X1.A60 | X2.A60 42.54,70 42.54,69.2 41.27,67.93 41.27,66.98 41.75,66.5 41.75,65.08 v40.96,64.28 40,63.33 40,55.39 40.32,55.07 40.32,51.58 v40.64,51.26 | v31.91,60.95 31.91,63.49 R6.1 | v28.57,60.95 27.62,60 27.62,58.25 27.94,57.93 27.94,53.49 27.62,53.17 v27.62,51.26 | v20.8,60.79 20.8,66.82 20.64,66.98 20.64,67.93 21.91,69.2 21.91,70 X3.A60
  Bottom 0.254: v61.59,65.08 61.28,65.39 50.48,65.39 50.16,65.08 50.16,64.28 49.05,64.28 48.74,64.6 41.27,64.6 v40.96,64.28 | v31.91,60.95 v28.57,60.95 26.67,60.95 26.35,60.63 20.95,60.63 v20.8,60.79 | v27.62,51.26 27.94,50.95 40.32,50.95 v40.64,51.26
RES  (via drill 0.3)
  Top 0.254: X2.A11 45.08,132.39 45.08,134.77 X2.A9 44.93,134.77 44.61,134.45 43.34,134.45 43.02,134.77 42.07,134.77 40.96,133.66 v40.96,133.5 | X2.B10 37.46,133.5 37.46,132.7 36.19,131.43 36.19,130.48 37.46,129.21 37.46,128.58 X2.B14
  Bottom 0.254: v40.96,133.5 37.46,133.5 X2.B10
RES.  (via drill 0.3)
  Top 0.254: X3.A41 24.45,94.13 24.45,93.65 22.38,91.59 21.43,91.59 20.64,92.38 20.64,93.33 21.91,94.6 21.91,95.4 X3.A40 | X3.A11 24.45,132.39 24.45,134.77 X3.A9 24.29,134.77 23.97,134.45 22.7,134.45 22.38,134.77 21.43,134.77 v20.48,133.81 | v14.45,133.5 v14.45,128.42 | v26.83,94.13 26.51,94.13 26.51,103.18 26.67,103.33 26.67,110.95 26.83,111.11 26.83,111.27 26.67,111.43 26.67,115.72 26.51,115.88 26.51,118.1 26.83,118.42 26.83,123.34 26.67,123.5 26.67,123.65 26.83,123.81 v26.83,131.43 26.83,131.75 26.67,131.91 26.67,139.53 26.51,139.69 26.51,149.53 26.99,150.01 v26.99,150.64 | X1.A11 65.72,132.39 65.72,134.77 X1.A9 65.56,134.93 64.45,134.93 64.29,135.08 63.82,135.08 63.5,134.77 62.71,134.77 v61.59,133.66 | 56.59,130.72 56.51,130.8 v56.51,133.5 | 56.59,130.72 58.1,129.21 58.1,128.58 X1.B14 | X2.A41 44.93,94.29 44.13,94.29 43.81,94.6 42.54,94.6 42.54,95.4 X2.A40 | v56.51,130.16 56.51,130.64 56.59,130.72 | v53.5,130.16 53.82,129.85 53.82,126.51 53.5,126.19 53.5,112.54 53.02,112.07 53.02,110.32 52.86,110.16 v52.86,94.6 | v46.67,151.12 46.99,151.44 46.99,159.69 46.67,160.01 v46.67,163.66 | v70.48,162.39 70.48,150.64 70.17,150.32 70.17,143.66 70.48,143.34 v70.48,138.74
  Bottom 0.254: v14.45,128.42 16.67,128.42 X3.B14 | v14.45,133.5 16.67,133.5 X3.B10 16.83,133.5 19.84,133.5 20.16,133.81 v20.48,133.81 | v26.83,94.13 24.45,94.13 X3.A41 | v26.83,131.43 26.51,131.75 25.88,131.75 25.4,132.23 24.45,132.23 X3.A11 | v56.51,133.5 57.94,133.5 X1.B10 58.1,133.5 60.96,133.5 61.12,133.66 v61.59,133.66 | 64.69,94.52 63.82,95.4 63.18,95.4 X1.A40 | 64.69,94.52 65.09,94.13 65.56,94.13 X1.A41 | 52.86,94.92 56.83,94.92 57.63,94.13 58.58,94.13 59.21,93.49 59.53,93.49 60.17,92.86 60.96,92.86 62.55,94.44 64.61,94.44 64.69,94.52 | 52.86,94.92 47.47,94.92 46.67,94.13 45.08,94.13 X2.A41 | v53.5,130.16 v56.51,130.16 | 52.86,94.92 v52.86,94.6 | v26.99,150.64 27.3,150.32 42.7,150.32 43.02,150.64 46.04,150.64 46.51,151.12 v46.67,151.12 | v46.67,163.66 49.05,163.66 49.69,163.02 60.8,163.02 61.75,162.07 70.17,162.07 v70.48,162.39 | v70.48,138.74 70.48,135.08 66.99,135.08 66.67,134.77 65.72,134.77 X1.A9
RST#  (via drill 0.3)
  Top 0.254: v74.61,127.15 v74.61,140.96
  Bottom 0.152: X6.J3-D28 87.36,140.96 80.01,140.96
  Bottom 0.254: X3.A15 24.45,127.15 38.26,127.15 39.53,128.42 40.48,128.42 41.75,127.15 44.93,127.15 X2.A15 45.08,127.15 58.9,127.15 60.17,125.88 60.96,125.88 62.23,127.15 65.56,127.15 X1.A15 65.72,127.15 v74.61,127.15 | v74.61,140.96 80.01,140.96
SERR#  (via drill 0.3)
  Top 0.203: v56.36,92.86 56.36,92.06 55.8,91.43 55.64,91.19 55.64,84.28 56.36,83.49
  Top 0.254: 56.36,83.49 v56.36,63.01 v56.36,57.3 | v35.08,63.01 35.08,83.49 34.77,83.81 34.77,92.54 v35.08,92.86 | v101.44,103.18 101.44,96.83 101.76,96.51 101.76,88.25 v101.44,87.94 | v105.41,87.94 105.09,87.94 105.09,77.46 105.41,77.14 105.41,73.97 106.04,73.33 106.04,70 106.36,69.68 106.36,46.5 106.68,46.18 v106.68,45.07 | v73.98,45.07 73.66,45.39 73.66,55.87 v73.98,56.19
  Bottom 0.152: X6.J3-A9 arc90 93.39,103.18 100.33,103.18
  Bottom 0.254: X2.B42 37.31,92.86 v35.08,92.86 23.65,92.86 22.38,91.59 21.43,91.59 20.16,92.86 16.83,92.86 X3.B42 | v56.36,92.86 57.94,92.86 X1.B42 | v56.36,63.01 56.04,63.33 48.42,63.33 48.1,63.65 42.23,63.65 41.59,63.01 v35.08,63.01 | v101.44,103.18 100.33,103.18 | v105.41,87.94 v101.44,87.94 | v106.68,45.07 105.57,45.07 105.25,45.39 82.39,45.39 82.07,45.07 v73.98,45.07 | v73.98,56.19 73.82,56.34 73.66,56.34 73.34,56.66 64.45,56.66 63.5,57.61 56.67,57.61 v56.36,57.3
STOP#  (via drill 0.3)
  Top 0.203: 56.51,90.48 56.12,90.08 56.12,84.52 56.83,83.81
  Top 0.254: v12.06,96.35 12.06,90 12.38,89.68 12.38,88.57 12.06,88.25 12.06,64.44 12.38,64.12 v12.38,57.3 | v46.51,68.25 46.83,67.93 46.83,66.35 46.51,66.03 46.51,60.47 46.83,60.15 v46.83,57.61 46.51,57.3 46.51,52.38 46.83,52.06 46.83,51.42 v46.99,51.26 | v49.53,68.25 49.53,76.66 49.85,76.98 49.85,81.74 50.16,82.06 | v57.15,82.22 56.83,82.54 56.83,83.81 | 56.51,90.48 57.63,91.59 58.42,91.59 59.37,92.54 59.37,94.6 59.69,94.92 v59.69,95.24 | v46.67,90.32 46.67,91.75 45.56,92.86 44.61,92.86 44.29,93.17 43.97,93.17 43.02,94.13 42.07,94.13 41.27,94.92 41.27,95.87 42.07,96.67 42.23,96.67 42.54,96.98 42.54,97.94 X2.A38 | v50.48,90.32 50.48,83.97 50.16,83.65 50.16,82.06 | 50.16,82.06 v50.32,82.06 | v103.82,107.14 103.82,89.84 103.19,89.21 103.19,84.76 102.87,84.44 102.87,80.79 103.19,80.47 103.19,76.19 103.5,75.87 103.5,72.7 104.14,72.06 104.14,70.95 102.87,69.68 102.87,57.14 v103.19,56.82 | v91.12,56.5 91.28,56.34 91.28,52.85 91.44,52.69 v91.44,49.99
  Bottom 0.152: X6.J3-A11 arc90 93.42,107.14 100.33,107.14
  Bottom 0.254: v12.06,96.35 16.03,96.35 16.35,96.67 17.3,96.67 18.57,97.94 21.75,97.94 X3.A38 | v12.38,57.3 30.64,57.3 30.96,57.61 v46.83,57.61 | v49.53,68.25 v46.51,68.25 | v50.32,82.06 50.64,81.74 56.51,81.74 56.99,82.22 v57.15,82.22 | v59.69,95.24 60.01,95.24 60.17,95.4 60.96,95.4 62.07,96.51 62.07,97.94 63.02,97.94 X1.A38 | v50.48,90.32 v46.67,90.32 | v103.82,107.14 100.33,107.14 | v103.19,56.82 102.08,56.82 101.76,56.5 v91.12,56.5 | v91.44,49.99 91.28,49.84 89.69,49.84 89.53,49.68 61.91,49.68 60.64,50.95 58.42,50.95 57.78,51.58 47.31,51.58 v46.99,51.26
TCK  (via drill 0.3)
  Top 0.254: v58.1,148.58 58.1,143.82 X1.B2 | v45.72,151.44 v45.72,148.58 | v37.31,151.12 37.31,145.4 37.46,145.24 37.46,143.82 X2.B2
  Bottom 0.254: X2.B2 37.31,143.66 23.65,143.66 22.38,142.39 21.43,142.39 20.16,143.66 16.83,143.66 X3.B2 | v58.1,148.58 57.78,148.9 46.04,148.9 v45.72,148.58 | v45.72,151.44 45.72,151.12 42.7,151.12 42.39,150.8 37.62,150.8 v37.31,151.12
TDI  (via drill 0.3)
  Top 0.254: v17.78,160.33 17.78,144.77 18.89,143.66 19.84,143.66 20.16,143.34 20.32,143.34 21.91,141.75 21.91,141.28 X3.A4 | v59.05,159.69 59.05,144.77 60.17,143.66 61.12,143.66 63.18,141.59 63.18,141.28 X1.A4 | v35.88,140.64 36.19,140.64 36.99,139.85 37.94,139.85 38.26,140.16 38.58,140.16 39.53,141.12 40.48,141.12 40.8,140.8 42.07,140.8 42.39,141.12 X2.A4
  Bottom 0.254: v17.78,160.33 24.45,160.33 25.08,159.69 33.97,159.69 34.61,159.06 55.4,159.06 56.04,159.69 v59.05,159.69 | v35.88,140.64 35.88,140.32 25.72,140.32 24.92,141.12 21.91,141.12 X3.A4
TDO  (via drill 0.3)
  Top 0.254: v15.24,150.17 15.24,149.05 14.92,148.74 14.92,143.82 16.83,141.91 16.83,141.28 X3.B4 | v24.92,148.1 v24.92,150.17 | X2.B4 37.46,141.28 37.46,142.07 36.04,142.07 35.88,142.23 35.88,147.47 v36.19,147.78 36.04,147.78 36.04,148.42 35.88,148.58 v35.88,152.23 | v47.94,141.59 47.62,141.91 47.62,149.21 47.94,149.53 47.94,150.32 48.26,150.64 v48.26,152.23
  Bottom 0.254: v15.24,150.17 15.56,149.85 22.38,149.85 22.7,150.17 v24.92,150.17 | v24.92,148.1 25.24,148.42 34.13,148.42 34.77,147.78 v36.19,147.78 | v47.94,141.59 48.26,141.91 55.56,141.91 56.36,141.12 57.94,141.12 X1.B4 | v35.88,152.23 v48.26,152.23
TMS
  Bottom 0.254: X3.A3 24.45,142.39 38.26,142.39 39.53,141.12 40.48,141.12 41.75,139.85 43.02,139.85 43.18,140.01 43.81,140.01 43.81,141.75 44.45,142.39 44.93,142.39 X2.A3 45.08,142.39 58.9,142.39 60.17,141.12 61.12,141.12 62.39,139.85 63.5,139.85 63.66,140.01 64.45,140.01 64.45,141.75 65.09,142.39 65.56,142.39 X1.A3
TRDY#  (via drill 0.3)
  Top 0.254: v10.79,98.89 10.79,88.57 11.11,88.25 11.11,64.44 10.79,64.12 v10.79,56.5 | v49.69,60.79 v49.69,56.82 | v94.46,61.11 94.46,76.19 94.77,76.51 v94.77,81.27 | v97.63,81.27 97.95,81.59 97.95,84.92 | 97.95,84.92 97.95,88.41 97.63,88.73 97.63,89.36 97.95,89.68 97.95,97.62 97.63,97.94 v97.55,110.2 | v64.61,102.86 63.18,101.43 63.18,100.64 X1.A36 | v72.55,85.87 v72.55,102.86 | 97.95,84.92 v97.63,84.92 | v46.35,105.87 45.88,105.87 45.56,105.56 44.61,105.56 44.29,105.24 43.97,105.24 43.02,104.29 42.07,104.29 41.27,103.49 41.27,102.54 42.54,101.27 42.54,100.64 X2.A36 | v48.42,103.49 v48.42,105.87 | v56.51,103.49 56.83,103.49 57.63,104.29 58.42,104.29 v59.53,105.4
  Bottom 0.152: X6.J3-B12 92.43,110.2 v97.55,110.2
  Bottom 0.254: v10.79,98.89 16.03,98.89 16.35,99.21 17.3,99.21 18.57,100.48 21.75,100.48 X3.A36 | v10.79,56.5 12.7,56.5 13.02,56.82 30.96,56.82 31.27,57.14 46.2,57.14 46.51,56.82 v49.69,56.82 | v49.69,60.79 50.01,60.47 67.94,60.47 68.58,61.11 78.42,61.11 78.74,60.79 85.72,60.79 86.04,61.11 v94.46,61.11 | v97.63,81.27 v94.77,81.27 | v64.61,102.86 65.09,102.86 65.17,102.94 | 65.17,102.94 65.25,103.02 66.2,103.02 66.36,102.86 v72.55,102.86 | v72.55,85.87 72.87,86.19 86.04,86.19 86.99,85.24 94.14,85.24 94.46,84.92 v97.63,84.92 | v48.42,105.87 v46.35,105.87 | v48.42,103.49 48.74,103.81 56.2,103.81 v56.51,103.49 | v59.53,105.4 59.69,105.56 61.28,105.56 62.55,104.29 63.82,104.29 65.17,102.94
TRST#
  Bottom 0.254: X3.A1 24.45,144.93 38.26,144.93 39.53,143.66 40.48,143.66 41.75,142.39 43.02,142.39 43.18,142.55 43.81,142.55 43.81,144.29 44.45,144.93 44.93,144.93 X2.A1 45.08,144.93 58.9,144.93 60.17,143.66 61.12,143.66 62.39,142.39 63.5,142.39 63.66,142.55 64.45,142.55 64.45,144.29 65.09,144.93 65.56,144.93 X1.A1
V3VAUX
  Bottom 0.254: X3.A14 21.91,128.42 35.72,128.42 36.99,129.69 37.94,129.69 39.21,130.96 40.48,130.96 40.64,130.8 41.27,130.8 41.27,129.69 42.39,128.58 X2.A14 42.54,128.42 56.36,128.42 57.63,129.69 58.58,129.69 59.85,128.42 63.02,128.42 X1.A14
V5P  (via drill 0.3)
  Top 0.152: X5.4 74.77,26.18 68.74,26.18 C13.1 68.58,26.18 61.44,26.18 R1.2
  Top 0.254: 89.06,43.49 X7.19 | 89.06,47.61 X7.20 | v81.76,22.37 81.44,22.69 81.44,26.18 | 81.44,26.18 81.44,30.31 v81.76,30.63 | v81.76,26.18 81.44,26.18 | v96.8,140.24 v96.84,137.15 v96.84,129.05 v96.84,128.18 | v85.25,142.27 v85.25,134.29 84.61,133.66 84.61,124.92 84.3,124.61 84.3,118.57 84.45,118.42 84.45,106.99 84.14,106.67 84.14,100.79 84.45,100.48 v84.45,89.21 | v67.31,139.85 v67.31,136.04 v67.31,134.29 | X1.B5 60.64,139.85 60.64,139.05 63.18,136.51 63.18,136.2 X1.A8 | X3.A5 24.45,139.85 24.45,139.05 21.91,136.51 21.91,136.2 X3.A8 | 42.54,136.51 42.54,136.83 v40.8,138.58 40,139.37 40,139.85 X2.B5 | 42.54,136.51 42.54,136.2 X2.A8 42.54,136.51 | 42.54,136.51 45.08,139.05 45.08,139.85 X2.A5 | v19.37,67.3 19.37,68.73 X3.B61 | v40,67.3 40,68.73 X2.B61 | v45.08,67.3 45.08,68.73 X2.A61 | v60.64,67.3 60.64,68.73 X1.B61 | v72.55,79.68 v72.55,72.54 v72.55,68.73 | v83.82,70.63 C9.+ 83.82,64.12 83.82,59.68 85.09,58.41 85.09,57.46 85.41,57.14 v85.41,47.61 | v75.09,70.63 75.09,72.38 JP3.3 | v78.74,81.74 v78.74,89.21 | v74.77,81.74 74.77,79.68 JP2.1
  Top 0.813: 89.06,47.61 89.06,43.49 | v85.41,30.79 v85.41,43.49
  Bottom 0.152: X6.J3-B27 91.36,140.16 92.23,140.16 92.63,140.16 92.63,140.2 v96.8,140.24 | X6.J3-C28 88.65,142.15 arc90 88.41,142.19 v85.25,142.27 | X6.J3-D2 v84.45,89.21 83.66,89.21 79.85,89.21 | X6.J3-A26 arc90 93.42,137.15 v96.84,137.15 | X6.J3-A22 arc90 93.52,129.05 v96.84,129.05 | X6.J3-C24 88.88,133.88 arc90 88.71,134.21 86.44,134.21 86.36,134.29 v85.25,134.29 81.28,134.29 | X6.J3-C1 88.65,87.92 arc90 88.39,88.17 88.07,88.17 88.07,88.25 83.66,88.17 | X6.J3-B21 91.36,127.85 arc-90 92.37,128.22 v96.84,128.18
  Bottom 0.254: v81.76,22.37 83.5,22.37 X7.4 | 81.91,30.79 v81.76,30.63 | 89.06,43.49 X7.19 | 74.93,26.18 X5.4 | 92.23,140.16 90.8,140.16 89.69,141.28 89.38,141.28 X6.J3-C28 | 59.29,139.13 60.01,139.85 60.48,139.85 X1.B5 | 59.29,139.13 58.74,138.58 58.1,138.58 X1.B6 | v67.31,136.04 63.18,136.04 X1.A8 | v67.31,139.85 65.72,139.85 X1.A5 | X3.A8 21.75,136.04 18.89,136.04 17.94,136.99 17.94,138.58 16.83,138.58 X3.B6 16.83,138.74 17.94,139.85 19.21,139.85 X3.B5 | v40.8,138.58 37.46,138.58 X2.B6 | X3.A5 24.45,139.85 39.85,139.85 X2.B5 | 59.29,139.13 59.21,139.21 58.74,139.21 58.58,139.37 51.75,139.37 51.43,139.05 47.47,139.05 46.67,139.85 45.08,139.85 X2.A5 | v67.31,134.29 81.28,134.29 | 19.37,67.46 21.75,67.46 X3.A62 21.91,67.46 37.31,67.46 X2.B62 37.46,67.46 40,67.46 | 19.37,67.46 16.83,67.46 X3.B62 | X3.B61 19.37,68.73 24.29,68.73 X3.A61 | v19.37,67.3 19.37,67.46 | 40,67.46 42.39,67.46 X2.A62 42.54,67.46 44.93,67.46 v45.08,67.3 45.08,67.46 57.94,67.46 X1.B62 58.1,67.46 60.64,67.46 | 40,67.46 v40,67.3 | 60.64,67.46 63.02,67.46 X1.A62 | X1.B61 60.64,68.73 65.56,68.73 X1.A61 65.72,68.73 v72.55,68.73 | v60.64,67.3 60.64,67.46 | 83.66,88.17 83.66,89.21 | v72.55,79.68 73.66,79.68 73.82,79.52 74.77,79.52 JP2.1 | v72.55,72.54 74.93,72.54 JP3.3 | v75.09,70.63 v83.82,70.63 | v78.74,89.21 79.85,89.21 | v74.77,81.74 v78.74,81.74 | 89.06,47.61 X7.20
  Bottom 0.813: 81.91,30.79 83.5,30.79 X7.6 83.66,30.79 v85.41,30.79 | v85.41,43.49 89.06,43.49 | 74.93,26.18 v81.76,26.18 | v85.41,47.61 89.06,47.61
V5VIO  (via drill 0.3)
  Top 0.254: X1.A10 63.18,133.5 63.18,132.7 64.45,131.43 64.45,128.1 63.18,126.83 63.18,126.04 X1.A16 63.18,125.88 63.18,125.08 64.45,123.81 64.45,123.5 v64.61,123.34 64.45,123.34 64.45,123.02 63.5,122.07 62.71,122.07 61.91,121.27 60.8,121.27 60.64,121.43 60.64,122.07 X1.B19 | v73.02,110.16 73.02,108.1 C15.1 | v68.1,123.34 68.1,119.21 67.79,118.89 67.79,113.18 68.1,112.86 v68.1,110.16 68.42,109.84 68.42,103.97 68.58,103.81 68.58,97.3 68.9,96.98 68.9,90 69.69,89.21 68.9,88.41 68.9,85.4 67.79,84.28 67.79,76.82 v68.1,76.51 68.42,76.19 68.42,71.58 v68.1,71.27 | 19.37,122.54 19.37,122.86 18.1,124.13 18.1,130.16 18.89,130.96 19.84,130.96 21.91,133.02 21.91,133.5 X3.A10 | 19.37,122.54 19.37,122.23 X3.B19 19.37,122.54 | 19.37,122.54 21.91,125.08 21.91,125.88 X3.A16 | X2.B19 40,122.23 40,122.86 42.54,125.4 42.54,125.88 X2.A16 42.54,126.04 42.54,126.67 43.81,127.94 43.81,131.43 42.54,132.7 42.54,133.5 X2.A10 | v26.03,126.35 26.35,126.67 26.35,130.8 26.03,131.12 26.03,133.97 v25.88,134.13 | v35.08,133.97 34.77,133.66 34.77,129.37 36.99,127.15 37.94,127.15 v38.89,126.19 | 44.13,71.58 44.45,71.58 44.93,72.06 45.08,72.06 45.08,71.43 X2.A59 45.08,71.27 45.08,70.63 v46.51,69.2 | 44.13,71.58 43.34,71.58 43.02,71.27 40,71.27 X2.B59 | v77.31,76.51 77.31,79.52 JP2.2 | v26.03,71.27 26.03,68.89 25.72,68.57 25.72,68.25 25.56,68.09 25.56,66.5 24.76,65.71 24.76,65.23 23.97,64.44 v23.97,54.6 | v36.35,58.41 v36.35,54.92 | v44.13,58.41 44.13,67.93 43.81,68.25 43.81,69.2 44.13,69.52 44.13,71.58 | v50.48,125.56 50.16,125.24 50.16,116.35 50.48,116.03 50.48,101.75 50.8,101.43 50.8,92.7 v50.48,92.38
  Top 0.254: v52.55,92.38 52.23,92.06 52.23,89.36 51.91,89.05 51.91,84.6 52.07,84.44 52.07,73.49 53.02,72.54 v53.02,69.2
  Bottom 0.254: v73.02,110.16 72.71,110.48 68.42,110.48 v68.1,110.16 | v64.61,123.34 v68.1,123.34 | v26.03,126.35 25.88,126.19 25.24,126.19 24.92,125.88 21.91,125.88 X3.A16 | v25.88,134.13 26.03,134.29 32.07,134.29 32.38,133.97 v35.08,133.97 | v38.89,126.19 39.21,126.19 39.53,125.88 42.39,125.88 X2.A16 42.54,125.88 45.56,125.88 45.88,125.56 v50.48,125.56 | X3.B59 19.37,71.43 20.32,72.38 20.32,73.01 20.64,73.01 21.43,73.81 22.38,73.81 23.49,72.7 23.49,71.27 24.29,71.27 X3.A59 24.45,71.27 v26.03,71.27 | v68.1,76.51 v77.31,76.51 | v68.1,71.27 65.72,71.27 X1.A59 65.56,71.27 60.64,71.27 X1.B59 60.48,71.27 59.69,71.27 59.69,70 58.42,68.73 57.63,68.73 56.83,69.52 53.02,69.52 | v46.51,69.2 46.83,69.52 53.02,69.52 | v23.97,54.6 24.29,54.92 v36.35,54.92 | v36.35,58.41 36.67,58.09 43.81,58.09 v44.13,58.41 | v52.55,92.38 v50.48,92.38 | 53.02,69.52 v53.02,69.2
V12M  (via drill 0.3)
  Top 0.152: X5.2 74.77,15.86 74.77,15.55 68.74,15.55 C11.1 68.58,15.39 60.8,15.39 R3.2
  Top 0.203: X3.B1 18.26,144.95 18.26,155.56 | X2.B1 38.73,146.18 38.73,153.82 39.69,154.77 39.85,154.77 | X1.B1 59.53,146.01 59.53,152.07 60.32,152.86 60.48,152.86 | X6.J3-A30 93.34,145.19 93.34,145.09 93.03,145.4 93.03,153.34
  Top 0.254: v96.36,145.24 96.04,144.93 96.04,136.83 96.36,136.51 96.36,129.69 95.57,128.89 95.57,111.75 95.25,111.43 95.25,105.87 95.57,105.56 95.57,80.95 95.25,80.63 v95.25,75.87 | v81.44,75.87 81.44,73.65 81.76,73.33 81.76,64.6 v81.44,64.28 | 59.53,152.07 59.53,159.06 59.85,159.37 v59.85,167.31 | 39.85,154.77 v39.85,167.79 | 18.26,155.56 18.26,159.69 18.57,160.01 v18.57,168.74 | v75.09,163.34 v75.09,168.26 | v93.03,163.66 93.03,162.55 92.71,162.23 92.71,153.66 93.03,153.34
  Top 0.813: v87.47,16.02 v87.47,13.96
  Bottom 0.152: X6.J3-A30 arc-90 93.39,145.24 v96.36,145.24 | X7.12 89.38,14.12 90.8,15.55 95.88,15.55 108.27,27.93 108.27,75.71 95.25,75.71 v95.25,75.87
  Bottom 0.254: 89.06,13.96 X7.12 | 74.93,16.02 X5.2 | v95.25,75.87 94.93,75.55 81.76,75.55 v81.44,75.87 | v81.44,64.28 78.26,64.28 C7.- | v18.57,168.74 18.89,168.42 25.56,168.42 25.88,168.1 27.15,168.1 27.46,167.79 28.26,167.79 28.57,167.47 40,167.47 v39.85,167.79 40.16,167.47 47.94,167.47 48.58,168.1 50.48,168.1 51.59,166.99 59.53,166.99 v59.85,167.31 59.69,166.99 63.18,166.99 63.82,167.63 72.39,167.63 72.71,167.95 73.5,167.95 73.82,168.26 v75.09,168.26 | v75.09,163.34 75.41,163.02 91.28,163.02 91.92,163.66 v93.03,163.66
  Bottom 0.813: v87.47,13.96 89.06,13.96 | 74.93,16.02 v87.47,16.02
V12P  (via drill 0.3)
  Top 0.152: R2.2 59.21,14.43 65.72,20.94 74.77,20.94 X5.3
  Top 0.254: v23.02,149.37 23.02,146.2 22.86,146.04 22.86,145.72 21.91,144.77 21.91,143.82 X3.A2 | v43.66,149.37 43.66,146.2 43.5,146.04 43.5,145.72 42.54,144.77 42.54,143.82 X2.A2 | v64.29,149.37 64.29,148.26 | 64.29,148.26 64.29,146.2 64.13,146.04 64.13,145.72 63.18,144.77 63.18,143.82 X1.A2 | v94.77,148.1 v94.77,143.18 | 64.29,148.26 v64.77,148.26 | v78.74,47.14 78.74,38.25 C12.1 78.74,38.09 v78.74,21.1 | 75.56,57.77 C8.+ | v68.9,148.26 68.9,133.18 68.58,132.86 68.58,123.97 68.9,123.65 68.9,123.02 68.58,122.7 68.58,118.89 68.26,118.57 68.26,113.49 68.9,112.86 68.9,104.29 69.06,104.13 69.06,97.62 69.37,97.3 69.37,90.32 70.17,89.52 70.17,88.73 69.37,87.94 v69.37,57.93
  Top 0.813: v75.56,47.14 75.56,57.77
  Bottom 0.152: X6.J3-A29 arc-90 93.49,143.34
  Bottom 0.254: v23.02,149.37 v43.66,149.37 v64.29,149.37 | v94.77,143.18 93.5,143.18 X6.J3-A29 | v94.77,148.1 94.46,147.78 83.82,147.78 83.34,148.26 v68.9,148.26 v64.77,148.26 | 83.34,47.14 X7.10 | v78.74,21.1 74.93,21.1 X5.3 | v69.37,57.93 C8.+
  Bottom 0.813: 83.34,47.14 v78.74,47.14 v75.56,47.14
V33  (via drill 0.3)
